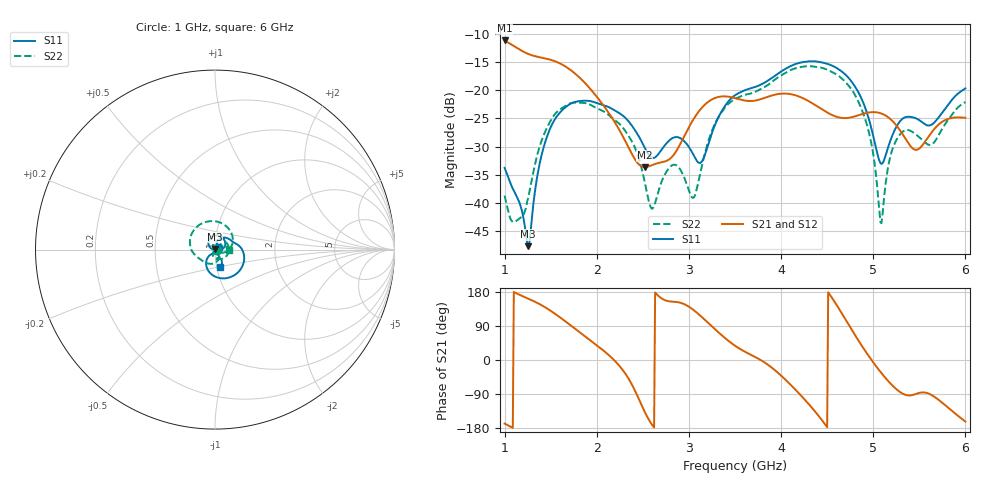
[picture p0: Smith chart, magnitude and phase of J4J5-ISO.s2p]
!Agilent Technologies,E8364B,MY43040528,A.07.50.67
!Agilent E8364B: A.07.50.67
!Date: Sunday, March 01, 2026 16:41:08
!Correction: S11(Full 2 Port(1,2))
!S21(Full 2 Port(1,2))
!S12(Full 2 Port(1,2))
!S22(Full 2 Port(1,2))
!S2P File: Measurements: S11, S21, S12, S22:
# Hz S  dB  R 50
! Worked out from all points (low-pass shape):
!   451 points, 1 GHz to 6 GHz, reference 50 ohm
!   highest |S21| = -11.19 dB at 1 GHz (marker M1); lowest = -33.6 dB at 2.522 GHz (marker M2)
!   |S21| within 3 dB of the highest: start of sweep to 1.391 GHz
!   lowest |S11| = -47.6 dB at 1.256 GHz (marker M3), VSWR 1.01, Z = 49.9 + j0.404 ohm
!   |S11| at or under -10 dB: start of sweep to end of sweep
!   |S22| runs from -43.6 to -15.7 dB; largest |S21 - S12| = 0.0012
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1e9  -33.76 33.3  -11.19 -167.8  -11.23 -167.7  -38.68 -5.4
1.1e9  -37.78 42.7  -12.17 179.5  -12.20 179.5  -43.36 27.3
1.255556e9  -47.64 102.9  -13.58 161.9  -13.62 161.9  -39.14 103.8
1.477778e9  -27.44 144.8  -14.51 133.3  -14.54 133.4  -26.07 79.6
1.844444e9  -21.88 75.7  -18.26 67.8  -18.29 67.9  -22.24 -7.9
2.288889e9  -24.59 19.5  -28.36 -28.8  -28.39 -28.7  -26.76 -91.4
2.522222e9  -30.24 8.0  -33.63 -137.8  -33.68 -137.7  -36.40 -122.2
2.6e9  -31.97 22.5  -33.27 -171.1  -33.31 -171.0  -41.01 -91.6
2.666667e9  -31.35 35.8  -32.92 169.6  -32.95 169.7  -38.05 -61.5
2.844444e9  -28.35 33.8  -31.24 153.6  -31.29 153.6  -33.20 -82.0
3.055556e9  -31.65 27.0  -24.98 130.9  -25.02 130.9  -38.97 -64.8
3.266667e9  -26.81 73.4  -21.50 85.0  -21.54 85.0  -26.51 -56.8
3.5e9  -20.90 47.3  -21.40 37.7  -21.44 37.8  -21.60 -108.1
4.344444e9  -14.87 -44.7  -22.37 -128.8  -22.41 -128.8  -15.79 109.2
4.844444e9  -20.55 -122.0  -24.41 49.4  -24.45 49.5  -22.23 -0.2
4.977778e9  -26.62 -133.5  -23.90 1.2  -23.94 1.3  -29.29 -28.3
5.077778e9  -32.90 -103.1  -24.08 -31.1  -24.12 -31.1  -43.38 8.5
5.166667e9  -29.85 -60.7  -24.85 -56.7  -24.89 -56.7  -33.14 73.5
5.3e9  -25.33 -64.4  -27.34 -86.0  -27.38 -85.9  -27.66 49.6
5.466667e9  -25.00 -78.6  -30.56 -89.4  -30.61 -89.4  -27.89 20.5
5.644444e9  -26.00 -67.2  -27.23 -94.1  -27.28 -94.1  -29.51 26.6
6e9  -19.68 -73.2  -24.89 -162.3  -24.93 -162.3  -22.10 -3.5
